| TEXAS INSTRUMENTS ILVCR2245A_IOORPORATED
| Standard Linear and Logic Group
| IBIS Model of SN74LVCR2245A
| OCTAL BUS TRANSCEIVER WITH 3-STATE OUTPUTS
| This file contains package information for the following:
|  SSOP 20-pin (DB) package as [Component] LVCR2245A_DB
|  TVSOP 20-pin (DGV) package as [Component] LVCR2245A_DGV
|  SOIC 20-pin (DW) package as [Component] LVCR2245A_DW
|  SOP 20-pin (NS) package as [Component] LVCR2245A_NS
|  TSSOP 20-pin (PW) package as [Component] LVCR2245A_PW
|  QFN 20-pin (RGY) package as [Component] LVCR2245A_RGY
|  VFBGA 20-pin (GQN) package as [Component] LVCR2245A_GQN
| This device can be powered at the following Vccs:
|  1.8 volt Vcc
|  2.5 volt Vcc
|  3.3 volt Vcc
| This file provides unique models under the [Model Selector] for each Vcc.
| For operation at a specific Vcc, select the appropriate model after each
| [Model Selector] keyword.
[IBIS Ver]   3.2
[Comment char]  |_char
[File Name]   sn74lvcr2245a.ibs
[File Rev]   1.1 | e_die
[Date]   February 10, 2003
[Source]   Data created from TI-SPICE simulations at TI-SLL.
[Notes]   The following is an IBIS list for the LVCR2245A.
   Please contact sll ibis@ti.com with questions and
   comments LVCR2245A_IO concerning SLL IBIS models.
   This IBIS model is created from a BA (back annotated
   netlist).
   - Due to the fact that the device is 5-V input/output
   tolerant, the pullup data has some non-monotonic warnings.
   - Power-clamp data has been deleted since there is no
   power-clamp diode in the device.
[Disclaimer] Property of Texas Instruments Corporated.Unauthorized
   reproduction and/or distribution is strictly prohibited.
   This product is protected under copyright law.
   Created  2003, (C) Copyright  2003, Texas Instruments,Inc,
   All Rights Reserved
   UNLESS THERE IS A SIGNED, WRITTEN AGREEMENT TO THE
   CONTRARY, TEXAS INSTRUMENTS (TI) IS PROVIDING THE IBIS
   MODELS  AND WITHOUT ANY WARRANTY, EXPRESSED OR
   IMPLIED.  TI assumes no liability for:
   1) the accuracy of the IBIS models provided to your
   company;
   2) the proper fuLVCR2245A_IOtioning of these IBIS Models
   in your design or for any resulting applications; or
   3) infringement of patents, copyrights or intellectual
   property rights resulting from your use of these IBIS
   models.
   TI provides IBIS Models as a service to our customers.
   You and your company shall not distribute, sell or give
   these models to anyone else without prior written
   permission from TI.
   TI reserves the right to make changes to our products or
   to discontinue any semiconductor product or service
   without notice, and advises our customers to obtain the
   latest version of relevant information to verify, before
   placing orders, that the information being relied on is
   current.
   Please be aware that your receipt and use of the IBIS
   information provided shall serve as acceptaLVCR2245A_IOe
   of these terms and conditions.  If you do not accept these
   terms,you should return or destroy the IBIS models and any
   other accompanying information immediately.
| Component LVCR2245A_DB 20-pin SSOP
[Component]   LVCR2245A_DB
[Manufacturer]   Texas Instruments, ILVCR2245A_IO.
[Package]
|   typ   min   max
R_pkg   4.000e-02   3.500e-02   5.100e-02
L_pkg   3.495e-09   3.035e-09   4.314e-09
C_pkg   4.200e-13   3.460e-13   5.020e-13
[Pin]   signal_name   model_name   R_pin   L_pin   C_pin
1   DIR   LVCR2245A_DIR   4.900e-02   4.310e-09   5.020e-13
2   A1   LVCR2245A_IO   4.800e-02   3.903e-09   4.870e-13
3   A2   LVCR2245A_IO   3.500e-02   3.189e-09   3.960e-13
4   A3   LVCR2245A_IO   3.500e-02   3.036e-09   3.470e-13
5   A4   LVCR2245A_IO   3.500e-02   3.035e-09   3.670e-13
6   A5   LVCR2245A_IO   3.500e-02   3.035e-09   3.670e-13
7   A6   LVCR2245A_IO   3.500e-02   3.036e-09   3.470e-13
8   A7   LVCR2245A_IO   3.500e-02   3.189e-09   3.970e-13
9   A8   LVCR2245A_IO   4.700e-02   3.899e-09   4.880e-13
10   GND   GND   5.100e-02   4.314e-09   5.000e-13
11   B8   LVCR2245A_IO   5.100e-02   4.314e-09   5.000e-13
12   B7   LVCR2245A_IO   4.700e-02   3.899e-09   4.880e-13
13   B6   LVCR2245A_IO   3.500e-02   3.189e-09   3.970e-13
14   B5   LVCR2245A_IO   3.500e-02   3.036e-09   3.460e-13
15   B4   LVCR2245A_IO   3.500e-02   3.035e-09   3.670e-13
16   B3   LVCR2245A_IO   3.500e-02   3.035e-09   3.670e-13
17   B2   LVCR2245A_IO   3.500e-02   3.036e-09   3.460e-13
18   B1   LVCR2245A_IO   3.500e-02   3.189e-09   3.970e-13
19   NOE   LVCR2245A_OE   4.700e-02   3.899e-09   4.880e-13
20   VCC   POWER   5.100e-02   4.314e-09   5.020e-13
| Component LVCR2245A_DGV 20-pin TVSOP
[Component]   LVCR2245A_DGV
[Manufacturer]   Texas Instruments, ILVCR2245A_IO.
[Package]
|   typ   min   max
R_pkg   4.400e-02   3.800e-02   4.800e-02
L_pkg   2.561e-09   2.236e-09   2.961e-09
C_pkg   3.420e-13   2.640e-13   4.460e-13
[Pin]   signal_name   model_name   R_pin   L_pin   C_pin
1   DIR   LVCR2245A_DIR   4.400e-02   2.935e-09   4.170e-13
2   A1   LVCR2245A_IO   4.200e-02   2.869e-09   4.460e-13
3   A2   LVCR2245A_IO   4.300e-02   2.399e-09   3.160e-13
4   A3   LVCR2245A_IO   4.400e-02   2.236e-09   2.650e-13
5   A4   LVCR2245A_IO   4.600e-02   2.278e-09   2.640e-13
6   A5   LVCR2245A_IO   4.500e-02   2.274e-09   2.640e-13
7   A6   LVCR2245A_IO   4.400e-02   2.285e-09   2.690e-13
8   A7   LVCR2245A_IO   4.300e-02   2.452e-09   3.200e-13
9   A8   LVCR2245A_IO   4.400e-02   2.900e-09   4.460e-13
10   GND   GND   4.400e-02   2.961e-09   4.180e-13
11   B8   LVCR2245A_IO   4.500e-02   2.954e-09   4.180e-13
12   B7   LVCR2245A_IO   4.200e-02   2.847e-09   4.430e-13
13   B6   LVCR2245A_IO   4.500e-02   2.453e-09   3.190e-13
14   B5   LVCR2245A_IO   4.500e-02   2.297e-09   2.690e-13
15   B4   LVCR2245A_IO   4.800e-02   2.334e-09   2.680e-13
16   B3   LVCR2245A_IO   4.800e-02   2.335e-09   2.670e-13
17   B2   LVCR2245A_IO   4.600e-02   2.299e-09   2.680e-13
18   B1   LVCR2245A_IO   4.600e-02   2.457e-09   3.200e-13
19   NOE   LVCR2245A_OE   4.300e-02   2.848e-09   4.410e-13
20   VCC   POWER   3.800e-02   2.812e-09   4.080e-13
| Component LVCR2245A_DW 20-pin SOIC
[Component]   LVCR2245A_DW
[Manufacturer]   Texas Instruments, ILVCR2245A_IO.
[Package]
|   typ   min   max
R_pkg   3.800e-02   3.300e-02   4.500e-02
L_pkg   5.012e-09   4.110e-09   6.349e-09
C_pkg   7.170e-13   5.300e-13   8.680e-13
[Pin]   signal_name   model_name   R_pin   L_pin   C_pin
1   DIR   LVCR2245A_DIR   4.200e-02   6.336e-09   8.650e-13
2   A1   LVCR2245A_IO   4.300e-02   5.542e-09   8.670e-13
3   A2   LVCR2245A_IO   3.400e-02   4.714e-09   7.320e-13
4   A3   LVCR2245A_IO   3.400e-02   4.377e-09   5.910e-13
5   A4   LVCR2245A_IO   3.600e-02   4.130e-09   5.330e-13
6   A5   LVCR2245A_IO   3.500e-02   4.111e-09   5.300e-13
7   A6   LVCR2245A_IO   3.400e-02   4.284e-09   5.830e-13
8   A7   LVCR2245A_IO   3.400e-02   4.634e-09   7.260e-13
9   A8   LVCR2245A_IO   4.000e-02   5.518e-09   8.650e-13
10   GND   GND   4.300e-02   6.349e-09   8.660e-13
11   B8   LVCR2245A_IO   4.100e-02   6.281e-09   8.610e-13
12   B7   LVCR2245A_IO   4.500e-02   5.561e-09   8.680e-13
13   B6   LVCR2245A_IO   3.300e-02   4.778e-09   7.420e-13
14   B5   LVCR2245A_IO   3.500e-02   4.414e-09   5.960e-13
15   B4   LVCR2245A_IO   3.500e-02   4.110e-09   5.330e-13
16   B3   LVCR2245A_IO   3.600e-02   4.130e-09   5.330e-13
17   B2   LVCR2245A_IO   3.400e-02   4.377e-09   5.910e-13
18   B1   LVCR2245A_IO   3.400e-02   4.714e-09   7.310e-13
19   NOE   LVCR2245A_OE   4.300e-02   5.569e-09   8.680e-13
20   VCC   POWER   4.200e-02   6.308e-09   8.640e-13
| Component LVCR2245A_GQN 20-pin VFBGA
[Component]   LVCR2245A_GQN
[Manufacturer] Texas Instruments, ILVCR2245A_IO.
[Package]
|   typ   min   max
R_pkg   4.300e-02   3.300e-02   6.100e-02
L_pkg   1.317e-09   8.960e-10   2.088e-09
C_pkg   1.130e-13   6.400e-14   1.900e-13
[Pin]   signal_name   model_name   R_pin   L_pin   C_pin
A2   DIR   LVCR2245A_DIR   3.800e-02   1.199e-09   1.210e-13
A1   A1   LVCR2245A_IO   4.000e-02   1.067e-09   1.020e-13
B3   A2   LVCR2245A_IO   6.100e-02   1.999e-09   1.900e-13
B1   A3   LVCR2245A_IO   3.300e-02   9.630e-10   7.100e-14
C2   A4   LVCR2245A_IO   4.900e-02   1.523e-09   1.230e-13
C1   A5   LVCR2245A_IO   3.300e-02   8.960e-10   6.400e-14
D3   A6   LVCR2245A_IO   6.100e-02   1.899e-09   1.640e-13
D1   A7   LVCR2245A_IO   3.300e-02   8.980e-10   6.700e-14
E2   A8   LVCR2245A_IO   4.900e-02   1.514e-09   1.280e-13
E1   GND   GND   3.600e-02   1.006e-09   9.400e-14
E3   B8   LVCR2245A_IO   4.900e-02   1.683e-09   1.460e-13
E4   B7   LVCR2245A_IO   3.300e-02   1.121e-09   8.900e-14
D2   B6   LVCR2245A_IO   6.100e-02   2.088e-09   1.730e-13
D4   B5   LVCR2245A_IO   3.300e-02   1.027e-09   7.100e-14
C3   B4   LVCR2245A_IO   4.900e-02   1.558e-09   1.240e-13
C4   B3   LVCR2245A_IO   3.300e-02   9.280e-10   6.700e-14
B2   B2   LVCR2245A_IO   6.100e-02   1.921e-09   1.770e-13
B4   B1   LVCR2245A_IO   3.300e-02   9.010e-10   7.700e-14
A4   NOE   LVCR2245A_OE   3.700e-02   9.900e-10   9.800e-14
A3   VCC   POWER   3.500e-02   1.168e-09   1.190e-13
| Component LVCR2245A_NS 20-pin SOP
[Component]   LVCR2245A_NS
[Manufacturer]   Texas Instruments, ILVCR2245A_IO.
[Package]
|   typ   min   max
R_pkg   4.400e-02   2.900e-02   5.800e-02
L_pkg   3.666e-09   2.317e-09   5.115e-09
C_pkg   5.480e-13   3.160e-13   7.250e-13
[Pin]   signal_name   model_name   R_pin   L_pin   C_pin
1   DIR   LVCR2245A_DIR   5.800e-02   5.115e-09   7.250e-13
2   A1   LVCR2245A_IO   5.300e-02   4.591e-09   7.240e-13
3   A2   LVCR2245A_IO   4.900e-02   3.754e-09   5.720e-13
4   A3   LVCR2245A_IO   2.900e-02   2.549e-09   3.880e-13
5   A4   LVCR2245A_IO   3.100e-02   2.317e-09   3.160e-13
6   A5   LVCR2245A_IO   3.100e-02   2.317e-09   3.160e-13
7   A6   LVCR2245A_IO   2.900e-02   2.556e-09   3.990e-13
8   A7   LVCR2245A_IO   4.900e-02   3.754e-09   5.790e-13
9   A8   LVCR2245A_IO   5.300e-02   4.591e-09   7.240e-13
10   GND   GND   5.800e-02   5.115e-09   7.250e-13
11   B8   LVCR2245A_IO   5.800e-02   5.115e-09   7.250e-13
12   B7   LVCR2245A_IO   5.300e-02   4.591e-09   7.240e-13
13   B6   LVCR2245A_IO   4.900e-02   3.754e-09   5.790e-13
14   B5   LVCR2245A_IO   2.900e-02   2.557e-09   3.990e-13
15   B4   LVCR2245A_IO   3.100e-02   2.317e-09   3.160e-13
16   B3   LVCR2245A_IO   3.100e-02   2.317e-09   3.160e-13
17   B2   LVCR2245A_IO   2.900e-02   2.557e-09   3.990e-13
18   B1   LVCR2245A_IO   4.900e-02   3.754e-09   5.790e-13
19   NOE   LVCR2245A_OE   5.300e-02   4.591e-09   7.240e-13
20   VCC   POWER   5.800e-02   5.115e-09   7.250e-13
| Component LVCR2245A_PW 20-pin TSSOP
[Component]   LVCR2245A_PW
[Manufacturer]   Texas Instruments, ILVCR2245A_IO.
[Package]
|   typ   min   max
R_pkg   5.000e-02   4.200e-02   6.000e-02
L_pkg   2.802e-09   2.248e-09   3.553e-09
C_pkg   3.170e-13   2.020e-13   4.430e-13
[Pin]   signal_name   model_name   R_pin   L_pin   C_pin
1   DIR   LVCR2245A_DIR   5.500e-02   3.461e-09   4.400e-13
2   A1   LVCR2245A_IO   5.500e-02   3.150e-09   4.010e-13
3   A2   LVCR2245A_IO   4.200e-02   2.619e-09   3.020e-13
4   A3   LVCR2245A_IO   4.500e-02   2.273e-09   2.020e-13
5   A4   LVCR2245A_IO   4.500e-02   2.248e-09   2.240e-13
6   A5   LVCR2245A_IO   4.500e-02   2.273e-09   2.260e-13
7   A6   LVCR2245A_IO   4.400e-02   2.323e-09   2.050e-13
8   A7   LVCR2245A_IO   4.600e-02   2.704e-09   3.070e-13
9   A8   LVCR2245A_IO   6.000e-02   3.265e-09   4.110e-13
10   GND   GND   5.700e-02   3.506e-09   4.360e-13
11   B8   LVCR2245A_IO   5.800e-02   3.553e-09   4.370e-13
12   B7   LVCR2245A_IO   5.800e-02   3.193e-09   4.050e-13
13   B6   LVCR2245A_IO   4.200e-02   2.704e-09   3.110e-13
14   B5   LVCR2245A_IO   4.600e-02   2.392e-09   2.100e-13
15   B4   LVCR2245A_IO   4.700e-02   2.334e-09   2.290e-13
16   B3   LVCR2245A_IO   4.700e-02   2.300e-09   2.270e-13
17   B2   LVCR2245A_IO   4.700e-02   2.349e-09   2.070e-13
18   B1   LVCR2245A_IO   4.500e-02   2.677e-09   3.060e-13
19   NOE   LVCR2245A_OE   6.000e-02   3.235e-09   4.060e-13
20   VCC   POWER   5.600e-02   3.487e-09   4.430e-13
| Component LVCR2245A_RGY 20-pin QFN
[Component]   LVCR2245A_RGY
[Manufacturer]   Texas Instruments, ILVCR2245A_IO.
[Package]
|   typ   min   max
R_pkg   4.600e-02   3.500e-02   5.800e-02
L_pkg   1.131e-09   8.800e-10   1.396e-09
C_pkg   1.650e-13   1.420e-13   1.750e-13
[Pin]   signal_name   model_name   R_pin   L_pin   C_pin
1   DIR   LVCR2245A_DIR   5.300e-02   1.289e-09   1.420e-13
2   A1   LVCR2245A_IO   5.800e-02   1.386e-09   1.720e-13
3   A2   LVCR2245A_IO   4.600e-02   1.111e-09   1.730e-13
4   A3   LVCR2245A_IO   3.900e-02   9.650e-10   1.610e-13
5   A4   LVCR2245A_IO   3.500e-02   8.810e-10   1.650e-13
6   A5   LVCR2245A_IO   3.500e-02   8.800e-10   1.650e-13
7   A6   LVCR2245A_IO   3.900e-02   9.610e-10   1.610e-13
8   A7   LVCR2245A_IO   4.500e-02   1.105e-09   1.720e-13
9   A8   LVCR2245A_IO   5.800e-02   1.386e-09   1.720e-13
10   GND   GND   5.600e-02   1.352e-09   1.590e-13
11   B8   LVCR2245A_IO   5.300e-02   1.287e-09   1.550e-13
12   B7   LVCR2245A_IO   5.800e-02   1.396e-09   1.720e-13
13   B6   LVCR2245A_IO   4.700e-02   1.129e-09   1.750e-13
14   B5   LVCR2245A_IO   4.000e-02   9.760e-10   1.640e-13
15   B4   LVCR2245A_IO   3.500e-02   8.840e-10   1.690e-13
16   B3   LVCR2245A_IO   3.500e-02   8.810e-10   1.680e-13
17   B2   LVCR2245A_IO   3.900e-02   9.670e-10   1.620e-13
18   B1   LVCR2245A_IO   4.600e-02   1.118e-09   1.740e-13
19   NOE   LVCR2245A_OE   5.800e-02   1.396e-09   1.750e-13
20   VCC   POWER   5.200e-02   1.276e-09   1.440e-13
| Model LVCR2245A_DIR
[Model Selector]   LVCR2245A_DIR
LVCR2245A_DIR_18   1.8 volt Vcc
LVCR2245A_DIR_25   2.5 volt Vcc
LVCR2245A_DIR_33   3.3 volt Vcc
| Model LVCR2245A_OE
[Model Selector]   LVCR2245A_OE
LVCR2245A_OE_18   1.8 volt Vcc
LVCR2245A_OE_25   2.5 volt Vcc
LVCR2245A_OE_33   3.3 volt Vcc
| Model LVCR2245A_IO
[Model Selector]   LVCR2245A_IO
LVCR2245A_IO_18   1.8 volt Vcc
LVCR2245A_IO_25   2.5 volt Vcc
LVCR2245A_IO_33   3.3 volt Vcc
| Models and submodels in the file (9): LVCR2245A_DIR_18 (Input), LVCR2245A_DIR_25 (Input), LVCR2245A_DIR_33 (Input), LVCR2245A_OE_18 (Input), LVCR2245A_OE_25 (Input), LVCR2245A_OE_33 (Input), LVCR2245A_IO_18 (I/O), LVCR2245A_IO_25 (I/O), LVCR2245A_IO_33 (I/O)
